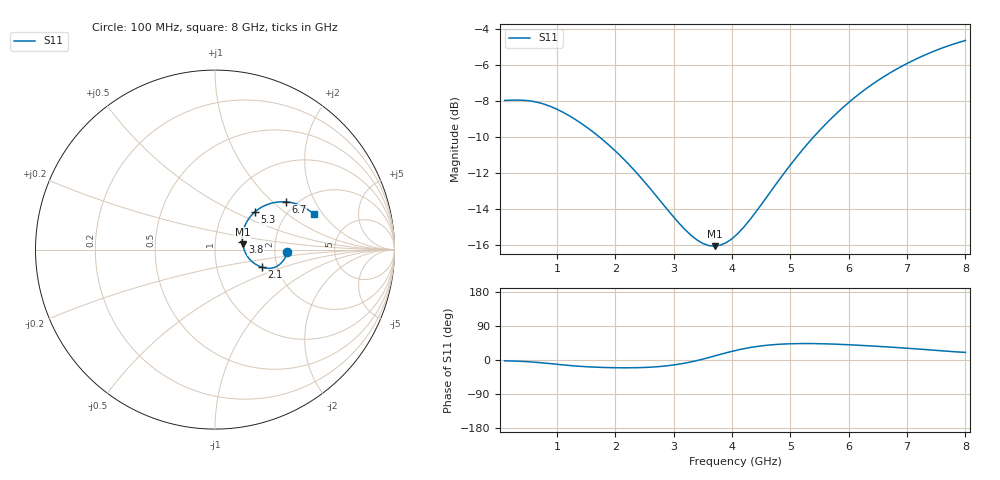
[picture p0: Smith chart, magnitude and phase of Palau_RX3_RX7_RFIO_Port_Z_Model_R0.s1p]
! Created Fri Jul 17 10:58:42 2020
! Palau RX3/RX7 RFIO Port Impedance Model.
! Revision		: R0.
! Impedance Mode 	: Balanced Differential-Mode.
! Impedance Format 	: Series Equivalent Differential Impedance (SEDZ).
# hz S ma R 50
! 1 Port Network Data from SP1.SP block
! freq  magS11  angS11
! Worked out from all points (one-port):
!   80 points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, 100 MHz to 8 GHz, reference 50 ohm
!   lowest |S11| = -16.1 dB at 3.7 GHz (marker M1), VSWR 1.37, Z = 68.1 + j4.06 ohm
!   |S11| at or under -10 dB: 1.72 GHz to 5.4 GHz (3.68 GHz wide, 103 % of centre)
!   S11 on the Smith chart (normalised r, x): 100 MHz: 2.32, -0.08; 2.1 GHz: 1.66, -0.35; 3.8 GHz: 1.36, +0.11; 5.3 GHz: 1.39, +0.64; 6.7 GHz: 1.76, +1.21; 8 GHz: 2.71, +1.65
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1e8  0.3988 -2.1
4e8  0.3994 -3.6
6e8  0.396 -5.6
8e8  0.3884 -8.3
1.1e9  0.3699 -12.8
1.3e9  0.3542 -15.6
1.6e9  0.3276 -18.5
1.8e9  0.3085 -19.7
2.1e9  0.2785 -20.5
2.6e9  0.2267 -18.9
3.1e9  0.1814 -10.7
3.4e9  0.1635 -1.4
3.6e9  0.1578 6.5
3.7e9  0.1572 10.7
3.8e9  0.1582 14.9
3.9e9  0.1608 19.0
4.1e9  0.1705 26.5
4.3e9  0.1857 32.7
4.6e9  0.2159 39.0
5.1e9  0.2771 43.2
5.3e9  0.3031 43.4
5.7e9  0.3553 42.1
6.1e9  0.406 39.5
6.4e9  0.4417 36.9
6.7e9  0.4746 34.1
7.1e9  0.5144 30.0
7.6e9  0.5573 24.2
8e9  0.5849 20.0
